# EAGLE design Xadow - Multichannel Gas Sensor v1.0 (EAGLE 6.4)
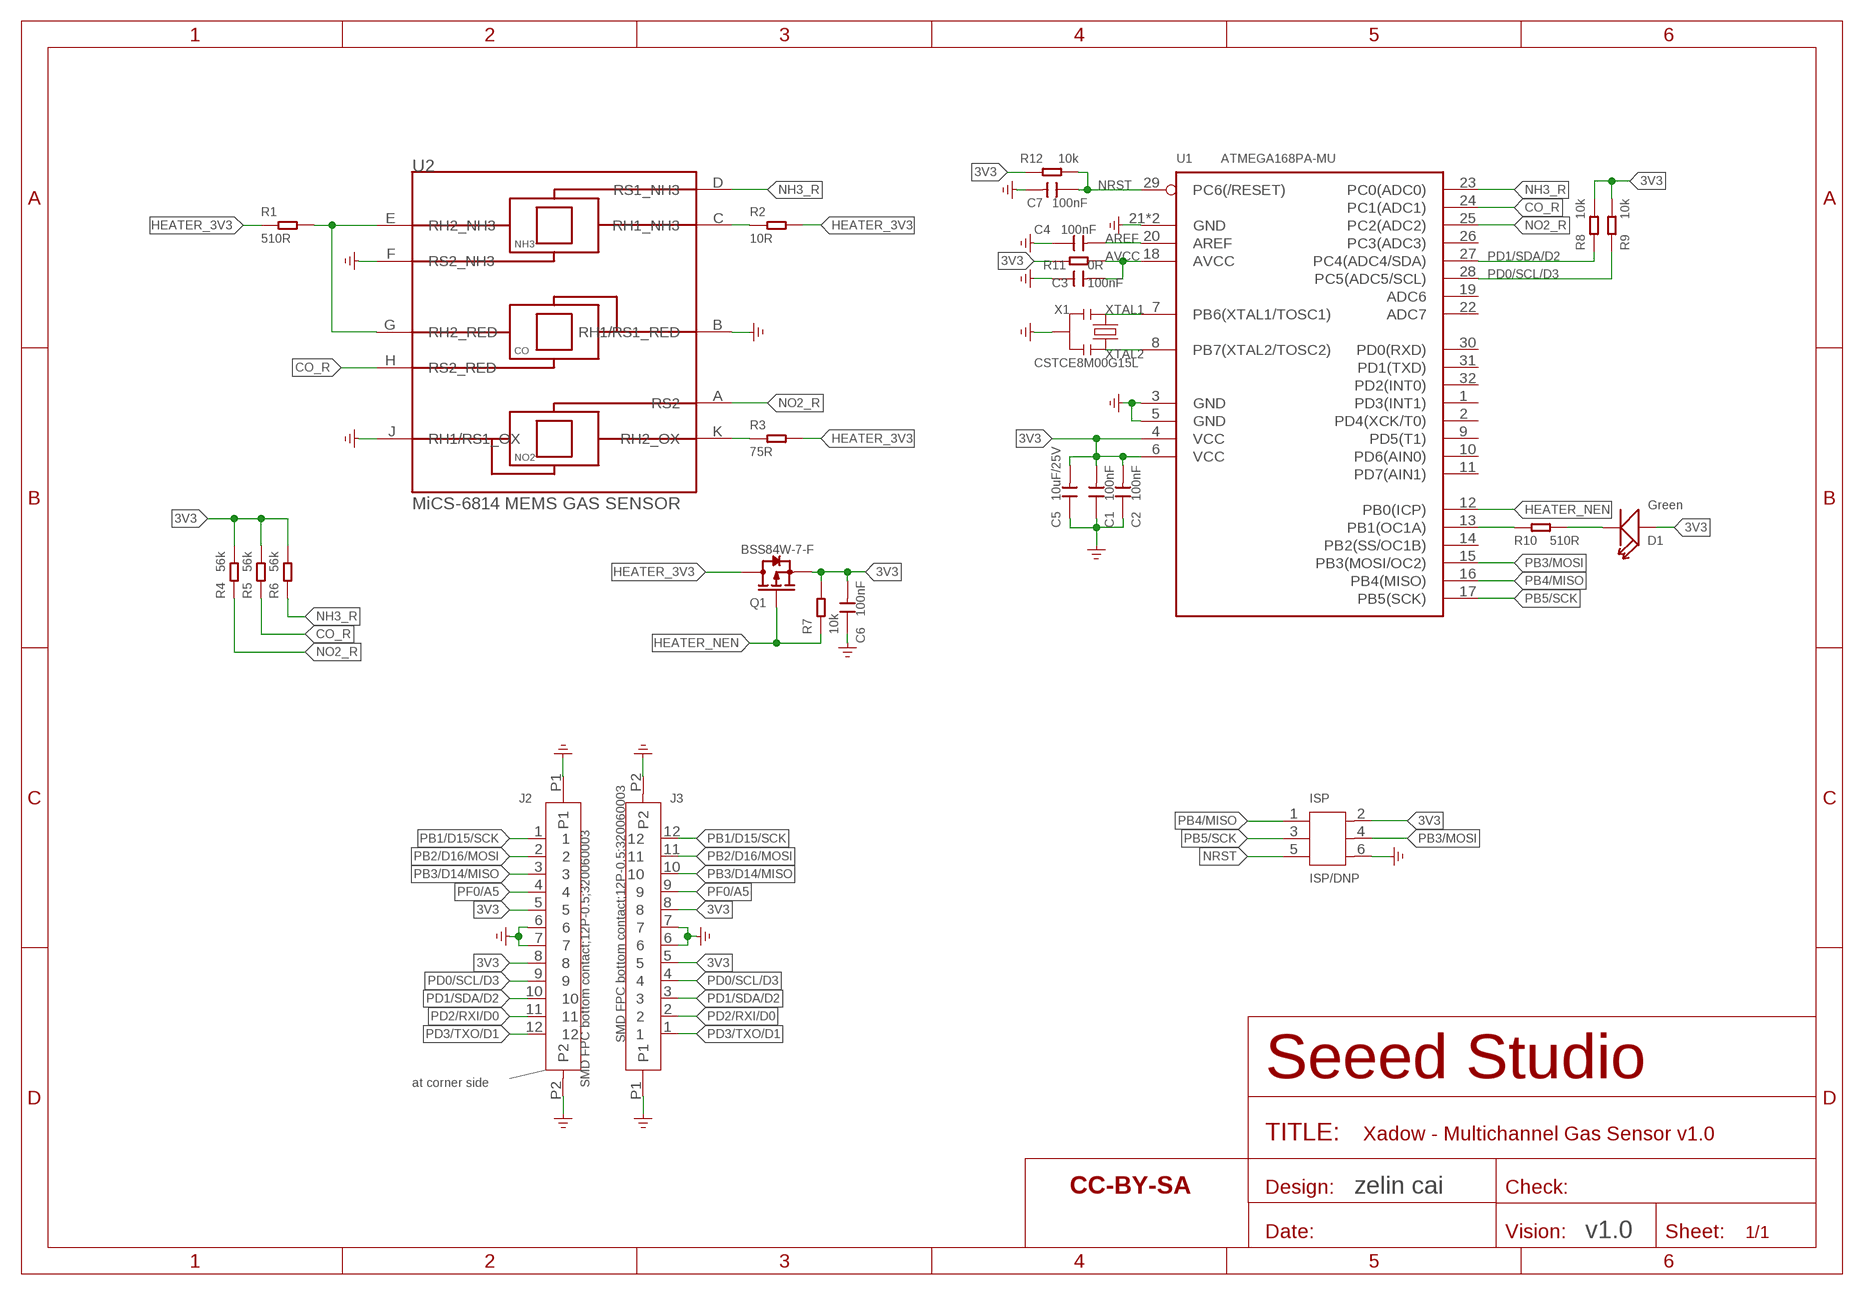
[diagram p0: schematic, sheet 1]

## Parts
C1  100nF  CAP-0402  [C0402]
C2  100nF  CAP-0402  [C0402]
C3  100nF  CAP-0402  [C0402]
C4  100nF  CAP-0402  [C0402]
C5  10uF/25V  CAP-0805  [C0805]
C6  100nF  CAP-0402  [C0402]
C7  100nF  CAP-0402  [C0402]
D1  Green  LED'0402'  [LED-0402]
ISP  ISP/DNP  HEADER-2X3P-1.27  [2X3P-1.27]
J2  SMD FPC bottom contact;12P-0.5;320060003  FPC-CONNECTOR-12P-FH12-12S-0.5SH  [12P-0.5]
J3  SMD FPC bottom contact;12P-0.5;320060003  FPC-CONNECTOR-12P-FH12-12S-0.5SH  [12P-0.5]
Q1  BSS84W-7-F  MOSFET-P-SOT323  [SOT-323]
R1  510R  RES-0402  [R0402]
R2  10R  RES-0402  [R0402]
R3  75R  RES-0402  [R0402]
R4  56k  RES-0402  [R0402]
R5  56k  RES-0402  [R0402]
R6  56k  RES-0402  [R0402]
R7  10k  RES-0402  [R0402]
R8  10k  RES-0402  [R0402]
R9  10k  RES-0402  [R0402]
R10  510R  RES-0402  [R0402]
R11  0R  RES-0402  [R0402]
R12  10k  RES-0402  [R0402]
U1  ATMEGA168PA-MU  MCU-ATMEGA8/168/328MU  [MLF-32]
U2  MiCS-6814  MICS-6814  [MICS-6814]
U$1  Xadow-Multichanel Gas Sensor  SEEEDSTUDIO-OPEN-SCH-FRAME  [SEEEDSTUDIO-PCB-FRAME]
X1  CSTCE8M00G15L  CRYSTAL-RESONATOR'SMD'  [3P-SMD-L3.6*W1.3MM]

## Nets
3V3: C1.2 C2.2 C5.2 C6.2 D1.+ ISP.2 J2.5 J2.8 J3.5 J3.8 Q1.2(S) R4.2 R5.2 R6.2 R7.2 R8.1 R9.1 R11.1 R12.2 U1.4(VCC) U1.6(VCC)
AREF: C4.2 U1.20(AREF)
AVCC: C3.2 R11.2 U1.18(AVCC)
CO_R: R5.1 U1.24(PC1(ADC1)) U2.H(RS2_RED)
GND: C1.1 C2.1 C3.1 C4.1 C5.1 C6.1 C7.2 ISP.6 J2.6 J2.7 J2.P1 J2.P2 J3.6 J3.7 J3.P1 J3.P2 U1.3(GND) U1.5(GND) U1.21(GND) U1.HEAT(GND) U2.B(RH1/RS1_RED) U2.F(RS2_NH3) U2.J(RH1/RS1_OX) X1.2 ; supply symbol labelled GND_POWER
HEATER_3V3: Q1.3(D) R1.1 R2.2 R3.2
HEATER_NEN: Q1.1(G) R7.1 U1.12(PB0(ICP))
N$1: R1.2 U2.E(RH2_NH3) U2.G(RH2_RED)
N$2: R2.1 U2.C(RH1_NH3)
N$3: R10.1 U1.13(PB1(OC1A))
N$4: R3.1 U2.K(RH2_OX)
N$5: D1.- R10.2
NH3_R: R6.1 U1.23(PC0(ADC0)) U2.D(RS1_NH3)
NO2_R: R4.1 U1.25(PC2(ADC2)) U2.A(RS2)
NRST: C7.1 ISP.5 R12.1 U1.29(PC6(/RESET))
PB1/D15/SCK: J2.1 J3.12
PB2/D16/MOSI: J2.2 J3.11
PB3/D14/MISO: J2.3 J3.10
PB3/MOSI: ISP.4 U1.15(PB3(MOSI/OC2))
PB4/MISO: ISP.1 U1.16(PB4(MISO))
PB5/SCK: ISP.3 U1.17(PB5(SCK))
PD0/SCL/D3: J2.9 J3.4 R9.2 U1.28(PC5(ADC5/SCL))
PD1/SDA/D2: J2.10 J3.3 R8.2 U1.27(PC4(ADC4/SDA))
PD2/RXI/D0: J2.11 J3.2
PD3/TXO/D1: J2.12 J3.1
PF0/A5: J2.4 J3.9
XTAL1: U1.7(PB6(XTAL1/TOSC1)) X1.1
XTAL2: U1.8(PB7(XTAL2/TOSC2)) X1.3
Unconnected: U1.1(PD3(INT1)) U1.2(PD4(XCK/T0)) U1.9(PD5(T1)) U1.10(PD6(AIN0)) U1.11(PD7(AIN1)) U1.14(PB2(SS/OC1B)) U1.19(ADC6) U1.22(ADC7) U1.26(PC3(ADC3)) U1.30(PD0(RXD)) U1.31(PD1(TXD)) U1.32(PD2(INT0))

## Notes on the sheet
- at corner side
- zelin cai
- v1.0

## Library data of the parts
C1-C4 C6 C7 = Discrete-new:CAP: Ceramic Capacitors; PN: 302010004
C5 = Discrete-new:CAP: Ceramic Capacitors; PN: 302010178
D1 = Discrete-new:LED; PN: 304090121
ISP = template:HEADER-2X3P-1.27
J2 J3 = Connector-new:FPC-CONNECTOR-12P: 320060003; PN: 320060003
Q1 = Discrete-new:MOSFET-P; PN: 305030012
R1 R10 = Discrete-new:RES; PN: 301010050
R2 = Discrete-new:RES; PN: 301010444
R3 = Discrete-new:RES; PN: 301010058
R4-R6 = Discrete-new:RES; PN: 301010032
R7-R9 R12 = Discrete-new:RES; PN: 301010047
R11 = Discrete-new:RES; PN: 301010000
U1 = IC-new:MCU-ATMEGA8/168/328; PN: 310010072
U2 = template:MICS-6814: SGX SensorTech MiCS-6814 MEMS Gas Sensor w/3 Indepedent Sensing Elements; PN: 314100015
U$1 = moudle-new:SEEEDSTUDIO-OPEN-SCH-FRAME
X1 = Discrete-new:CRYSTAL-RESONATOR: Resonator Small SMD resonator. This is the itty bitty 10/20MHz resonators with built in caps. CSTCE10M0G55 and CSTCE20M0V53. Footprint has been reviewed closely but hasn't been tested yet.; PN: 306030005

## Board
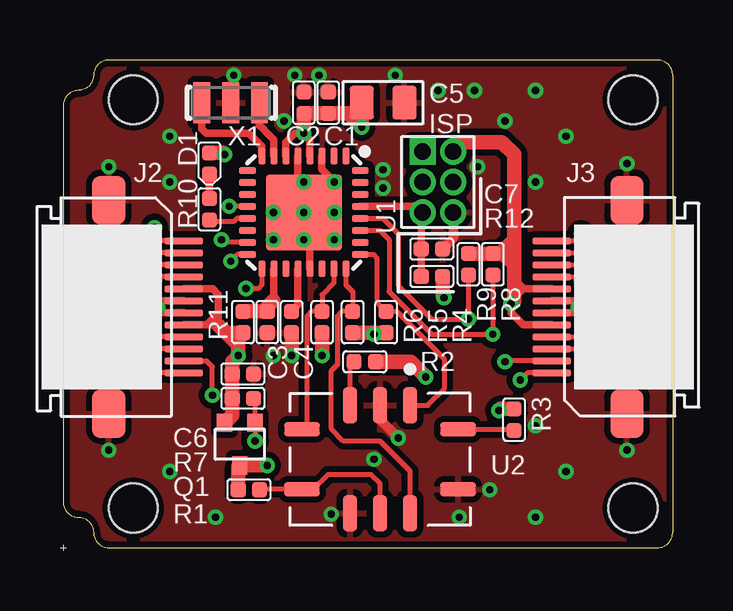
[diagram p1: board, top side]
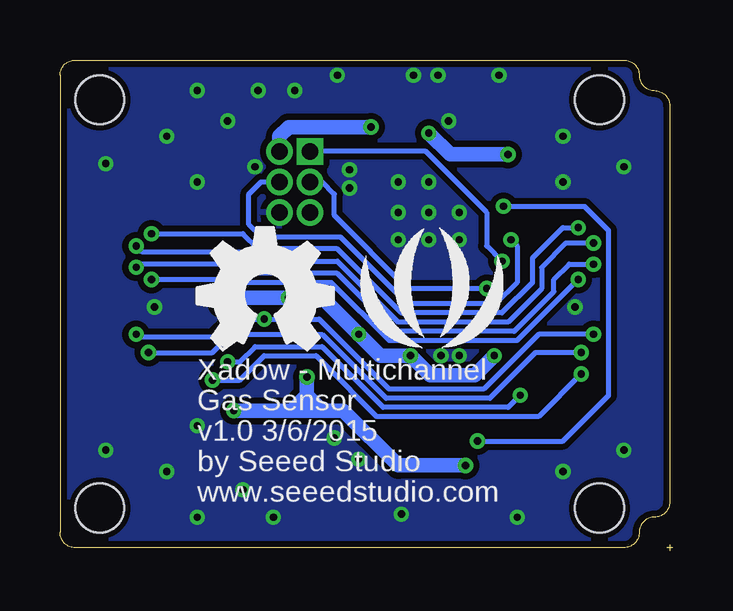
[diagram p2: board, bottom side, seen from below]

Size 25.53 x 20.45 mm. Coordinates in mm from the lower left corner, seen from the top.
Copper layers (1*16): Top 0.035mm / dielectric 1.5mm / Bottom 0.035mm
Design rules "SeeedStudio_2layer_DRU_no_angle_20140221 *": minimum track width 6mil, minimum drill 12mil, track to track 6mil, track to pad 6mil, pad to pad 6mil, via to via 6mil, smd to smd 0mil, copper to edge 10mil, drill to drill 10mil, minimum pad ring 6mil, minimum via ring 6mil, stop-mask expansion 2mil, vias tented up to drill 25mil, thermal gap 10mil

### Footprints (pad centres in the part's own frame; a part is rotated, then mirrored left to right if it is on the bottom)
C0402 = smd 0.635 x 0.635: 1 0,0.445; 2 0,-0.445
C0805 = smd 1.397 x 1.016: 1 0,0.889; 2 0,-0.889
LED-0402 = smd 0.635 x 0.635: + -0.445,0; - 0.445,0
2X3P-1.27 = drill 0.686 pad 1.092 square: 1 -0.635,1.27 | drill 0.686 pad 1.092: 2 0.635,1.27; 3 -0.635,0; 4 0.635,0; 5 -0.635,-1.27; 6 0.635,-1.27
12P-0.5 = smd 0.3 x 1.6: 1 -2.75,3.127; 2 -2.25,3.127; 3 -1.75,3.127; 4 -1.25,3.127; 5 -0.75,3.127; 6 -0.25,3.127; 7 0.25,3.127; 8 0.75,3.127; 9 1.25,3.127; 10 1.75,3.127; 11 2.25,3.127; 12 2.75,3.127 | smd 2.032 x 1.397: P1 -4.445,0; P2 4.445,0
SOT-323 = smd 0.635 x 0.762: 1 -0.635,-0.889; 2 0.635,-0.889; 3 0,0.889
R0402 = smd 0.635 x 0.635: 1 0,0.445; 2 0,-0.445
MLF-32 = smd 0.7 x 0.3: 1 -2.35,1.75; 2 -2.35,1.25; 3 -2.35,0.75; 4 -2.35,0.25; 5 -2.35,-0.25; 6 -2.35,-0.75; 7 -2.35,-1.25; 8 -2.35,-1.75; 17 2.35,-1.75; 18 2.35,-1.25; 19 2.35,-0.75; 20 2.35,-0.25; 21 2.35,0.25; 22 2.35,0.75; 23 2.35,1.25; 24 2.35,1.75 | smd 0.3 x 0.7: 9 -1.75,-2.35; 10 -1.25,-2.35; 11 -0.75,-2.35; 12 -0.25,-2.35; 13 0.25,-2.35; 14 0.75,-2.35; 15 1.25,-2.35; 16 1.75,-2.35; 25 1.75,2.35; 26 1.25,2.35; 27 0.75,2.35; 28 0.25,2.35; 29 -0.25,2.35; 30 -0.75,2.35; 31 -1.25,2.35; 32 -1.75,2.35 | smd 3.175 x 3.175: HEAT 0,0
MICS-6814 = smd 1.5 x 0.6: A 2.25,-1.25; B 2.25,0; C 2.25,1.25; F -2.25,1.25; G -2.25,0; H -2.25,-1.25 | smd 0.6 x 1.5: D 1.25,3.25; E -1.25,3.25; J -1.25,-3.25; K 1.25,-3.25
XADOW-DRILL-DIM-25*20MM = hole 2.032: -9.779,-8.509; -9.779,8.509; 11.049,8.509; 11.049,-8.509
3P-SMD-L3.6*W1.3MM = smd 0.7 x 1.7: 1 -1.2,0; 2 0,0; 3 1.2,0

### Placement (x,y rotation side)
C1  11.18,18.67 0 top
C2  10.16,18.67 0 top
C3  8.64,9.53 180 top
C4  9.65,9.53 180 top
C5  13.46,18.67 270 top
C6  7.62,7.37 270 top
C7  15.49,12.57 90 top
D1  6.22,16.13 270 top
ISP  15.75,15.37 0 top
J2  2.03,10.16 270 top
J3  23.62,10.16 90 top
Q1  7.49,4.45 180 top
R1  7.87,2.54 90 top
R2  12.7,7.87 90 top
R3  18.92,5.46 180 top
R4  13.59,9.53 0 top
R5  12.19,9.53 0 top
R6  10.92,9.53 0 top
R7  7.62,6.35 270 top
R8  18.03,11.94 0 top
R9  17.02,11.94 0 top
R10  6.22,14.22 180 top
R11  7.62,9.53 180 top
R12  15.49,11.43 90 top
U1  10.16,14.1 270 top
U2  13.34,3.81 90 top
U$1  not placed on the board
U$20  [XADOW-DRILL-DIM-25*20MM]  12.83,10.29 0 top
U$21  [OSHW_FILLX200_NOTEXT]  19.81,8.38 0 bottom
U$22  [SEEED-SILK-280*268MIL]  10.03,10.16 0 bottom
X1  7.11,18.67 180 top

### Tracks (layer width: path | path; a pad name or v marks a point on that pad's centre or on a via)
3V3  (via drill 0.3 pad 0.64)
  Top 0.305: U1.4 10.41,17.15 v10.16,17.4 9.78,17.4 9.41,17.03 U1.6 | J2.8 6.11,9.41 | 6.11,9.41 6.59,9.41 6.6,9.4 6.6,9.91 | J2.5 6.36,10.91 6.6,10.67 6.6,9.91 | 6.11,9.41 6.6,9.91 | J3.8 19.32,10.91 | 19.29,10.91 18.94,10.91 | J3.5 19.29,9.41 18.8,9.91 v18.8,10.29 | 19.32,10.91 18.92,11.3 | 19.32,10.91 19.29,10.91 | 19.29,10.91 18.92,10.54
  Top 0.61: D1.+ 6.8,16.57 v6.86,16.51 | R11.1 7.49,9.08 | 7.49,9.08 6.92,9.08 6.6,9.4 | 7.43,8.57 7.43,9.02 7.49,9.08 | 7.43,8.57 7.37,8.64 | 7.37,8.64 6.99,9.02 | 7.37,8.64 7.37,8.76 7.62,9.02 | R6.2 v10.92,8.13 | R9.1 R8.1 18.4,12.38 | 18.48,12.38 18.86,12.38 18.92,12.45 | 18.92,10.92 18.92,11.3 18.92,12.45 | 18.92,10.92 18.92,10.54 18.92,10.41 v18.8,10.29 | 18.94,10.91 18.92,10.92 | 7.43,8.57 v7.43,8.13 7.18,7.87 C6.2 R7.2 7.18,5.65 Q1.2 | R4.2 13.15,9.08 v13.08,9.02 13.02,9.08 R5.2 | 18.92,12.45 18.92,16.51 18.41,17.02 16.76,17.02 ISP.2 | 18.4,12.38 18.4,12.43 18.8,12.83 | 18.4,12.38 18.48,12.38 | 18.48,12.38 18.8,12.07 | R12.2 15.94,10.6 v16,10.54 | v10.16,17.4 C2.2 C1.2 12,18.23 v12.57,17.65 C5.2
  Bottom 0.61: v12.57,17.65 16,17.65 16.38,17.27 ISP.2 | v18.8,10.29 18.54,10.54 v16,10.54 14.61,10.54 v13.08,9.02 12.19,8.13 v10.92,8.13 10.1,7.3 8.26,7.3 v7.43,8.13 | v6.86,16.51 9.27,16.51 v10.16,17.4
AREF
  Top 0.305: U1.20 9.91,10.23 C4.2
AVCC
  Top 0.305: U1.18 8.91,10.43 8.89,10.41
  Top 0.61: 8.89,10.41 8.64,10.16 C3.2 R11.2
CO_R
  Top 0.203: U1.24 11.91,11.08 12.19,10.79 R5.1 11.75,9.97 11.56,9.78 11.56,7.75 11.3,7.49 11.3,5.08 11.81,4.57 13.34,4.57 14.59,3.32 U2.H
GND  (via drill 0.3 pad 0.64)
  Top 0.305: J2.6 4.31,10.41 v4.06,10.16 4.31,9.91 J2.7 | U1.5 9.91,15.62 v10.16,15.37 | U1.3 10.91,15.89 v11.43,15.37 | U1.21 10.41,12.7 v10.16,12.95 | J3.7 21.34,10.41 v21.59,10.16 21.34,9.91 J3.6
  Top 0.406: U2.B 13.34,5.46 v14.1,4.7 | ISP.6 16.38,13.02 C7.2
  Top 0.61: C4.1 v9.65,8.13
  other vias: 8.89,8.13 10.79,19.81 9.78,19.81 8.89,14.1 10.16,14.1 11.43,14.1 11.43,12.95 8.89,12.95 23.62,16.13 23.62,4.19 2.03,4.19 2.03,16 17.91,2.54 11.3,1.52 7.24,19.81 4.57,17.27 4.57,3.3 18.54,17.91 19.81,15.37 19.81,5.21 17.4,16 13.08,3.81 13.46,15.88 13.46,15.11 15.75,19.18 17.27,19.18 19.81,19.18 21.08,17.27 13.97,19.81 4.57,15.37 6.48,1.4 16.64,1.4 19.81,1.4 21.08,3.3 9.33,17.91
  pour Bottom (isolate 0.254, rank 6): -0.51,21.08 26.16,21.08 26.16,-0.51 -0.51,-0.51
  pour Top (isolate 0.254, rank 6): -0.51,21.08 26.16,21.08 26.16,-0.51 -0.51,-0.51
HEATER_3V3  (via drill 0.3 pad 0.64)
  Top 0.61: R2.2 14.61,7.87 v15.24,7.24 | v8.64,3.56 Q1.3 7.43,3.49 R1.1 | R3.2 18.35,5.91 v18.29,5.84
  Bottom 0.61: v8.64,3.56 11.43,3.56 13.72,5.84 14.61,5.84 | v18.29,5.84 15.88,5.84 | 15.88,5.84 15.24,5.84 | 15.24,5.84 14.61,5.84 | v15.24,7.24 15.24,6.48 | 15.24,6.48 15.24,5.84 | 15.24,6.48 14.61,5.84 | 15.24,6.48 15.88,5.84
HEATER_NEN  (via drill 0.3 pad 0.64)
  Top 0.203: U1.12 v7.05,14.35 | v8.13,4.57 Q1.1 8.13,6.29 R7.1
  Bottom 0.203: v8.13,4.57 4.57,4.57 2.67,6.48 2.67,13.34 3.68,14.35 v7.05,14.35
N$1
  Top 0.203: R1.2 8.34,2.56 U2.E 10.56,2.56 11.18,3.18 12.95,3.18 13.34,2.79 U2.G
N$2
  Top 0.203: U2.C 12.09,7.7 R2.1
N$3
  Top 0.203: U1.13 7.37,13.85 7.24,13.72 6.29,13.72 R10.1
N$4
  Top 0.203: U2.K 18.88,5.06 R3.1
N$5
  Top 0.305: R10.2 D1.-
NH3_R
  Top 0.203: U1.23 11.41,11.16 10.92,10.67 R6.1 10.48,9.97 10.29,9.78 10.29,5.26 U2.D
NO2_R
  Top 0.203: U1.25 13.05,12.35 13.21,12.19 13.21,10.35 R4.1 14.03,9.97 16,8 16,6.73 15.33,6.06 U2.A
NRST
  Top 0.305: U1.29 14.86,14.35 ISP.5 15.05,14.03 C7.1 R12.1
PB1/D15/SCK  (via drill 0.3 pad 0.64)
  Top 0.203: J3.12 21.42,12.91 v21.72,13.21 | J2.1 4.11,12.91 3.94,13.08 v3.94,13.46
  Bottom 0.203: v21.72,13.21 17.91,13.21 17.27,12.57 13.97,12.57 11.3,9.91 7.11,9.91 5.84,11.18 5.84,12.19 4.57,13.46 v3.94,13.46
PB2/D16/MOSI  (via drill 0.3 pad 0.64)
  Top 0.203: J2.2 3.97,12.41 3.56,12.83 v3.3,12.83 | J3.11 22.06,12.41 v22.35,12.7
  Bottom 0.203: v22.35,12.7 22.1,12.45 17.91,12.45 17.53,12.07 13.97,12.07 11.43,9.53 6.86,9.53 5.46,10.92 5.46,11.81 4.45,12.83 v3.3,12.83
PB3/D14/MISO  (via drill 0.3 pad 0.64)
  Top 0.203: J3.10 22.25,11.91 v22.35,11.81 | J2.3 3.33,11.91 v3.3,11.94
  Bottom 0.203: v3.3,11.94 4.32,11.94 4.95,11.3 4.95,10.79 6.6,9.14 11.56,9.14 13.97,11.56 17.65,11.56 18.03,11.94 22.23,11.94 v22.35,11.81
PB3/MOSI  (via drill 0.3 pad 0.64)
  Top 0.203: U1.15 6.84,12.85 v6.73,12.95
  Bottom 0.203: v6.73,12.95 6.48,12.7 6.48,11.18 7.37,10.29 11.05,10.29 13.84,13.08 17.15,13.08 17.65,13.59 17.65,14.86 17.15,15.37 ISP.4
PB4/MISO  (via drill 0.3 pad 0.64)
  Top 0.203: U1.16 7.39,12.35 v7.11,12.07
  Bottom 0.203: ISP.1 10.29,16.64 7.75,14.1 7.75,12.7 v7.11,12.07
PB5/SCK  (via drill 0.3 pad 0.64)
  Top 0.203: U1.17 8.41,11.08 8.26,10.92 v7.75,10.92
  Bottom 0.203: v7.75,10.92 11.05,10.92 14.1,13.97 14.1,14.86 14.61,15.37 ISP.3
PD0/SCL/D3  (via drill 0.3 pad 0.64)
  Top 0.203: U1.28 13.46,13.85 14.1,13.21 14.1,11.05 15.49,9.65 v17.02,9.65 R9.2 | J3.4 22.24,8.91 v22.35,9.02 | J2.9 3.41,8.91 v3.3,9.02
  Bottom 0.203: v22.35,9.02 22.23,8.89 19.18,8.89 18.41,9.65 v17.02,9.65 14.73,9.65 11.81,6.73 7.87,6.73 5.59,9.02 v3.3,9.02
PD1/SDA/D2  (via drill 0.3 pad 0.64)
  Top 0.203: U1.27 13.32,13.35 13.72,12.95 13.72,10.79 15.49,9.02 v18.03,9.02 R8.2 | J3.3 21.69,8.41 v21.84,8.26 | J2.10 3.97,8.41 v3.81,8.26
  Bottom 0.203: v21.84,8.26 19.18,8.26 18.41,9.02 v18.03,9.02 14.61,9.02 11.94,6.35 7.62,6.35 5.72,8.26 v3.81,8.26
PD2/RXI/D0  (via drill 0.3 pad 0.64)
  Top 0.203: J2.11 6.1,7.91 6.35,7.66 v6.35,6.48 | J3.2 18.58,7.91 v18.54,7.87
  Bottom 0.203: v18.54,7.87 18.03,7.87 17.4,8.51 14.61,8.51 12.07,5.97 6.86,5.97 v6.35,6.48
PD3/TXO/D1  (via drill 0.3 pad 0.64)
  Top 0.203: J2.12 3.85,7.41 v3.81,7.37 | J3.1 19.48,7.41 v19.18,7.11
  Bottom 0.203: v3.81,7.37 5.59,5.59 12.32,5.59 14.54,7.81 14.61,7.87 14.86,8.13 17.02,8.13 18.03,7.11 v19.18,7.11
PF0/A5  (via drill 0.3 pad 0.64)
  Top 0.203: J2.4 4.17,11.41 4.06,11.3 v3.94,11.3 | J3.9 21.61,11.41 v21.72,11.3
  Bottom 0.203: v21.72,11.3 18.29,11.3 18.16,11.18 14.22,11.18 11.81,8.76 6.48,8.76 v3.94,11.3
XTAL1
  Top 0.305: U1.7 8.91,17.12 8.64,17.4 8.44,17.6 8.31,17.72 X1.1
XTAL2
  Top 0.305: U1.8 8.41,16.86 7.87,17.4 6.1,17.4 5.91,17.58 X1.3

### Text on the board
bPlace: Xadow - Multichannel | Gas Sensor | v1.0 3/6/2015 | by Seeed Studio | www.seeedstudio.com

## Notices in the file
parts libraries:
moudle-new: This work is licensed under the Creative Commons Attribution 4.0 International License.
To view a copy of this license,visit:
http://creativecommons.org/licenses/by-sa/4.0
moudle-new: CC-BY-SA
